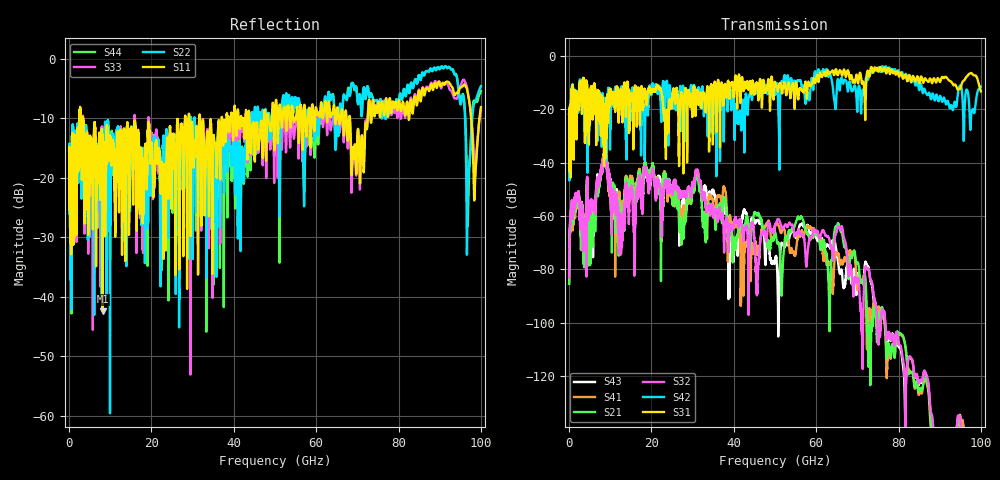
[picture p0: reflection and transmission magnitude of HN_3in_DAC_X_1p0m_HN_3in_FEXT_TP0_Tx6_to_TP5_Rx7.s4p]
# GHz S RI R 45
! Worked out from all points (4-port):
!   4000 points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, 25 MHz to 100 GHz, reference 45 ohm
!   strongest paths, dB at 25 MHz, 25.02 GHz, 50.02 GHz, 75.03 GHz, 100 GHz:
!     S31: -21.6, -16.6, -9.8, -5.2, -13.4
!     S42: -21.7, -14.4, -14.5, -5.1, -11.5
!     S32: -83.1, -50.7, -63.4, -106.8, -178.3
!     S21: -85.4, -51.8, -65.9, -99.8, -177.6
!     S41: -85.2, -52.8, -64.1, -96.0, -186.6
!     S43: -81.6, -50.5, -76.8, -99.4, -187.0
!   lowest |S11| = -42.4 dB at 8.175 GHz (marker M1), VSWR 1.02, Z = 45.6 + j0.333 ohm
!   |S11| at or under -10 dB: 3.377 GHz to 28.12 GHz (24.74 GHz wide, 157 % of centre); 31.8 GHz to 37.03 GHz (5.226 GHz wide, 15.2 % of centre); 68.23 GHz to 72.51 GHz (4.288 GHz wide, 6.09 % of centre)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
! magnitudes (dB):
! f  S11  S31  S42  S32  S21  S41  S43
! 25 MHz  -15.5  -21.6  -21.7  -83.1  -85.4  -85.2  -81.6
! 8.175 GHz  -42.4  -28.8  -13.9  -41.9  -41.3  -40.1  -41.3
! 12.55 GHz  -11.9  -14.2  -12.5  -59.8  -61.3  -71.1  -56.6
! 31.05 GHz  -11.8  -13.2  -15.6  -42.8  -45.8  -44.3  -43.5
! 39.02 GHz  -10.8  -15.5  -10.9  -64.8  -64.5  -60.3  -80.4
! 45.73 GHz  -12.6  -11.0  -12.6  -85.0  -59.3  -72.0  -61.8
! 100 GHz  -8.1  -13.4  -11.5  -178.3  -177.6  -186.6  -187.0
